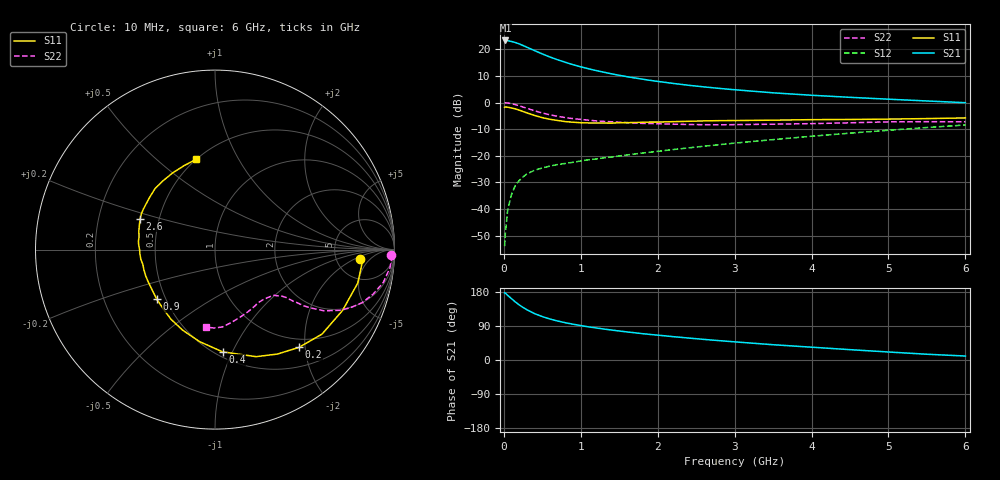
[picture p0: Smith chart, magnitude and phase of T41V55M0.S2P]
! Infineon Technologies  Discrete & RF Semiconductors
! BFR182T
! Si NPN RF Bipolar Junction Transistor in SC75
! VCE = 1.5 V  IC = 5 mA
! Common Emitter S-Parameters:  October  1999
# GHz  S  MA  R  50
!  f  S11  S21  S12  S22
! GHz  MAG  ANG  MAG  ANG  MAG  ANG  MAG  ANG
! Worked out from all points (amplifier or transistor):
!   36 points, 10 MHz to 6 GHz, reference 50 ohm
!   highest |S21| = 23.3 dB at 20 MHz (marker M1)
!   |S21| within 3 dB of that: start of sweep to 336 MHz
!   unconditionally stable (mu >= 1): 1.326 GHz to 4.093 GHz
!   at 250 MHz: K = 0.29, MSG = 24.7 dB, |S12| = -27.9 dB
!   at 1.4 GHz: K = 1.03, MAG = 14.6 dB, |S12| = -20.5 dB
!   at 6 GHz: K = 0.85, MSG = 4.2 dB, |S12| = -8.4 dB
!   lowest NFmin = 1.20 dB at 450 MHz
!   S11 on the Smith chart (normalised r, x): 10 MHz: 8.75, -2.76; 200 MHz: 0.84, -1.88; 400 MHz: 0.54, -0.92; 900 MHz: 0.45, -0.30; 2.6 GHz: 0.39, +0.17; 6 GHz: 0.50, +0.68
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0.01  0.8119 -3.8  14.54 177.4  0.002 80.7  0.9821 -1.9
0.02  0.8256 -4.0  14.66 176.5  0.0035 96.8  0.9865 -2.3
0.05  0.8169 -13.2  14.5 170.6  0.0096 86.2  0.9805 -5.8
0.1  0.7874 -25.5  14.02 161.8  0.0188 78.5  0.9553 -11.1
0.15  0.7597 -38.3  13.4 153.1  0.0278 70.8  0.9138 -15.9
0.2  0.7182 -49.3  12.64 145.4  0.0342 67.7  0.8709 -19.9
0.25  0.6782 -59.1  11.77 138.6  0.0401 62.5  0.8212 -23.2
0.3  0.639 -69.0  10.94 132.6  0.0456 59.7  0.7792 -25.7
0.4  0.5709 -85.8  9.448 122.3  0.0534 54.8  0.6971 -29.3
0.5  0.5198 -99.5  8.177 114.6  0.0589 52.2  0.6363 -31.0
0.6  0.4839 -111.8  7.153 108.1  0.064 51.0  0.5879 -32.3
0.7  0.4593 -122.2  6.352 102.9  0.0685 51.0  0.55 -32.8
0.9  0.4264 -139.6  5.134 94.4  0.0753 51.0  0.4978 -33.7
1.1  0.4133 -153.2  4.311 87.4  0.084 52.4  0.4656 -34.4
1.4  0.4102 -168.3  3.46 79.1  0.0946 54.3  0.4349 -36.3
1.6  0.4192 -177.0  3.059 74.1  0.1035 55.7  0.4179 -37.5
2.2  0.4369 166.1  2.286 61.6  0.1307 59.0  0.3928 -43.9
2.6  0.4514 157.5  1.966 54.4  0.151 60.1  0.3832 -49.0
3.5  0.4659 141.7  1.521 40.3  0.2008 60.3  0.3918 -61.8
4.5  0.4805 127.3  1.252 27.3  0.2656 57.5  0.4157 -77.1
5.5  0.499 110.0  1.069 15.2  0.3394 52.6  0.4368 -90.8
6  0.5138 101.7  0.993 10.5  0.3783 49.1  0.4343 -96.7
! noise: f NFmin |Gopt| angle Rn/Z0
0.45  1.2  0.27  37  0.3
0.9  1.3  0.25  75  0.23
1.8  1.9  0.21  145  0.2
